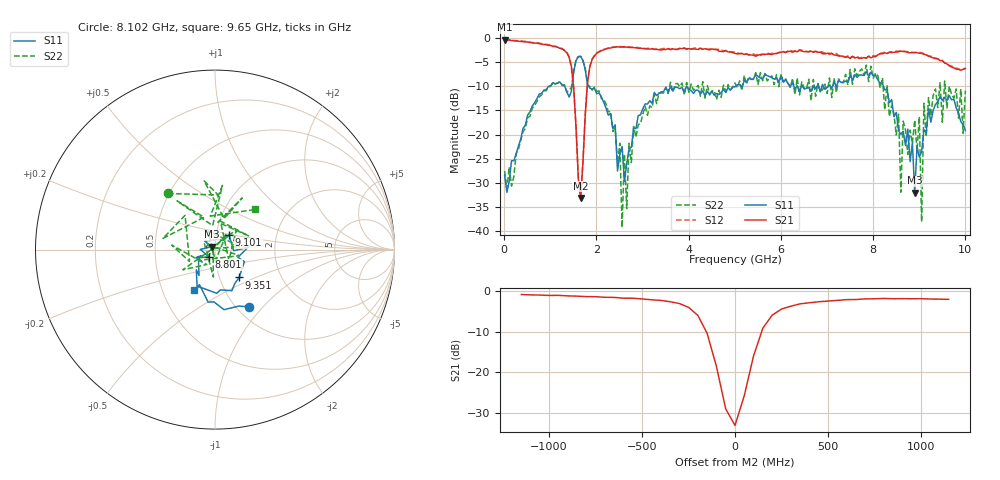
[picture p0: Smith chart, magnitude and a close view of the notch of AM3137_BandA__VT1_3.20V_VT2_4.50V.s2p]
! Date/Time: Tue, Nov 13, 2018 4:48 PM
! Network Analyzer: Agilent Technologies E8364B Rev: A.07.50.67
! Sweep from 0.010 to 10.000 GHz, 201 Points, Sweep Type: LIN
! Power Supply: 3.201 V, -0.003 A
# Hz S DB R 50
!freq MagS11 AngS11 MagS21 AngS21 MagS12 AngS12 MagS22 AngS22
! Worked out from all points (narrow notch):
!   201 points, 10 MHz to 10 GHz, reference 50 ohm
!   highest |S21| = -0.30 dB at 10 MHz (marker M1); lowest = -33.1 dB at 1.658 GHz (marker M2)
!   notch at M2: 30.3 dB deep, 193 MHz wide at half that depth
!   lowest |S11| = -32.1 dB at 8.901 GHz (marker M3), VSWR 1.05, Z = 48.2 + j1.61 ohm
!   |S11| at or under -10 dB: 1.835 GHz to 3.953 GHz (2.119 GHz wide, 73.2 % of centre); 3.961 GHz to 5.019 GHz (1.058 GHz wide, 23.6 % of centre); 8.224 GHz to end of sweep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
!   |S22| runs from -39.3 to -3.8 dB; largest |S21 - S12| = 0.032
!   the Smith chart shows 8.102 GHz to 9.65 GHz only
!   S11 on the Smith chart (normalised r, x): 8.102 GHz: 1.13, -0.84; 8.801 GHz: 0.93, -0.07; 9.101 GHz: 1.16, +0.19; 9.351 GHz: 1.24, -0.40; 9.65 GHz: 0.72, -0.35
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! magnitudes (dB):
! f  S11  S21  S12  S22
! 10 MHz  -28.5  -0.3  -0.2  -27.6
! 1.409 GHz  -12.2  -4.0  -3.9  -10.9
! 1.658 GHz  -3.8  -33.1  -32.9  -3.8
! 1.708 GHz  -4.6  -25.8  -25.8  -4.7
! 1.908 GHz  -10.5  -4.4  -4.3  -10.8
! 2.508 GHz  -24.2  -1.9  -1.7  -21.8
! 2.557 GHz  -22.5  -1.8  -1.8  -39.3
! 2.607 GHz  -29.7  -1.9  -1.8  -24.1
! 3.357 GHz  -11.5  -2.4  -2.3  -11.4
! 5.005 GHz  -10.1  -3.2  -2.9  -9.3
! 6.703 GHz  -9.9  -2.9  -2.8  -8.6
! 8.102 GHz  -8.6  -3.5  -3.5  -7.8
! 8.352 GHz  -13.4  -2.9  -2.9  -16.3
! 8.601 GHz  -20.0  -2.7  -2.7  -32.0
! 8.801 GHz  -25.6  -3.0  -2.9  -19.1
! 8.901 GHz  -32.1  -3.0  -3.0  -17.0
! 9.001 GHz  -24.7  -3.1  -3.0  -16.3
! 9.051 GHz  -23.6  -3.2  -3.0  -38.1
! 9.101 GHz  -19.0  -3.4  -3.3  -13.5
! 9.351 GHz  -13.8  -4.3  -4.1  -10.5
! 9.65 GHz  -11.9  -5.7  -5.7  -10.0
! 10 GHz  -19.2  -6.3  -6.2  -10.9
